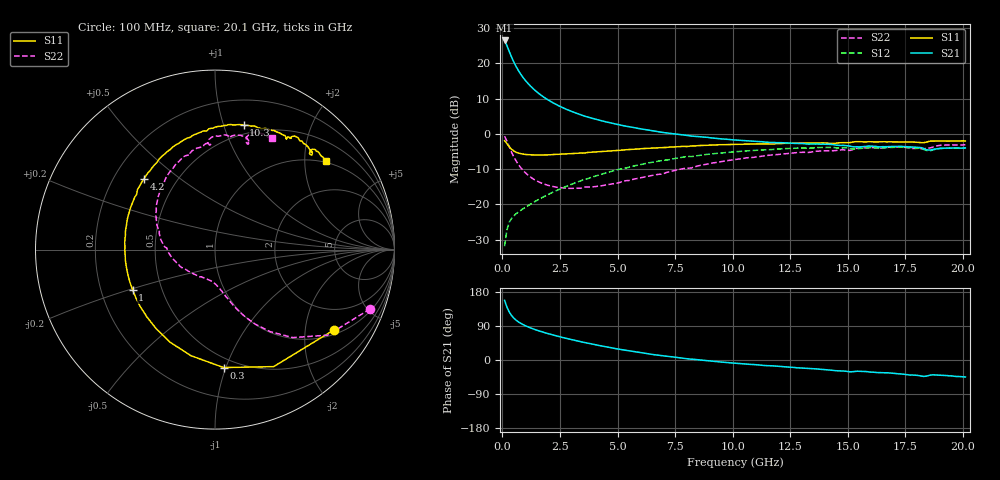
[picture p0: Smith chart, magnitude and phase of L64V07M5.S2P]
!  Infineon Technologies AG
! BFR380L3 , PF131585-7, No.6, Th 09.10.01, soldered on pcb-board, measured with PP GSG850
!  Vce=4.0 V,  Ic=7.5 mA
! Common Emitter S-Parameters:  15. November 2001
#  GHz  S  MA  R  50
! f  S11  S21  S12  S22
! GHz  Mag  Ang  Mag  Ang  Mag  Ang  Mag  Ang
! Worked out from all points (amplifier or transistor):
!   201 points, 100 MHz to 20.1 GHz, reference 50 ohm
!   highest |S21| = 26.5 dB at 100 MHz (marker M1)
!   |S21| within 3 dB of that: start of sweep to 292.9 MHz
!   unconditionally stable (mu >= 1): 2.013 GHz to 4.487 GHz
!   at 3.4 GHz: K = 1.03, MAG = 8.2 dB, |S12| = -13.3 dB
!   at 10.1 GHz: K = 0.94, MSG = 1.7 dB, |S12| = -5.1 dB
!   at 20.1 GHz: K = 0.99, MSG = 0.0 dB, |S12| = -4.0 dB
!   S11 on the Smith chart (normalised r, x): 100 MHz: 1.15, -2.87; 300 MHz: 0.42, -0.98; 1 GHz: 0.34, -0.21; 4.2 GHz: 0.33, +0.38; 10.3 GHz: 0.41, +1.17; 20.1 GHz: 0.96, +2.53
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0.1  0.8009 -33.8  21.04 157.4  0.02565 71.3  0.9253 -20.9
0.2  0.7294 -63.4  17.75 139.5  0.04359 61.1  0.788 -37.2
0.3  0.659 -85.8  14.69 126.7  0.05588 53.5  0.6551 -48.4
0.4  0.6059 -102.8  12.26 117.4  0.06308 49.3  0.5505 -56.1
0.5  0.5731 -116.0  10.39 110.4  0.06892 47.4  0.4718 -61.6
0.6  0.5491 -126.7  8.967 105.0  0.07385 46.7  0.4131 -65.7
0.7  0.5333 -135.4  7.874 100.5  0.07832 46.6  0.3674 -68.9
0.8  0.524 -142.5  6.997 96.7  0.08254 47.0  0.3321 -71.4
1  0.5106 -154.0  5.722 90.5  0.09105 48.3  0.2813 -75.6
1.2  0.5054 -162.9  4.834 85.3  0.1001 49.7  0.2478 -79.0
1.4  0.5031 -170.1  4.189 80.8  0.1093 51.1  0.2239 -82.2
1.9  0.5044 175.5  3.155 71.1  0.1339 53.4  0.1902 -90.0
2.6  0.5171 160.5  2.366 59.7  0.1708 54.4  0.1721 -102.2
3.5  0.5334 145.1  1.818 46.9  0.2221 52.9  0.1718 -118.3
4.2  0.5587 135.1  1.566 38.3  0.2617 50.8  0.1822 -133.6
5.2  0.588 122.7  1.314 27.1  0.3199 45.5  0.2108 -151.6
6.8  0.6366 104.9  1.07 12.2  0.4129 36.4  0.2674 179.3
10.1  0.7107 78.5  0.8185 -8.4  0.5573 14.5  0.4332 136.8
10.3  0.7126 77.1  0.8088 -9.3  0.5642 13.2  0.4418 134.4
13.5  0.7429 60.2  0.719 -23.0  0.6343 -7.6  0.5584 103.9
16.8  0.7726 47.9  0.6614 -34.1  0.6394 -24.4  0.6469 80.2
20.1  0.7905 38.6  0.6317 -44.8  0.63 -38.4  0.6995 62.8
